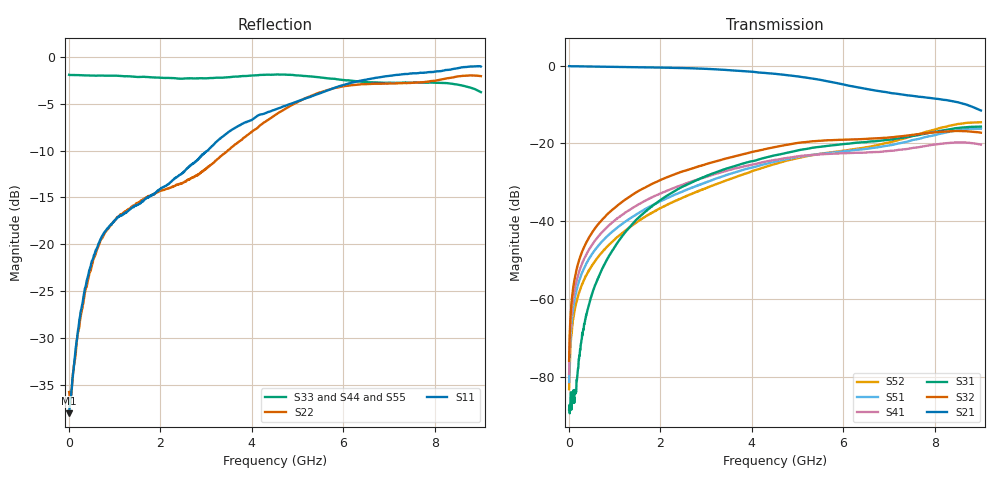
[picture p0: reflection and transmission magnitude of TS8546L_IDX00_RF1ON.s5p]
# GHz S DB R 50
! CMT, SN0916, 25263762, 26.7.0
! Date: 16.07.2026 08:25:07
! Data: Format
! Freq S1.1:dB/Ang S1.2:dB/Ang S1.3:dB/Ang S1.4:dB/Ang S1.5:dB/Ang
!  S2.1:dB/Ang S2.2:dB/Ang S2.3:dB/Ang S2.4:dB/Ang S2.5:dB/Ang
!  S3.1:dB/Ang S3.2:dB/Ang S3.3:dB/Ang S3.4:dB/Ang S3.5:dB/Ang
!  S4.1:dB/Ang S4.2:dB/Ang S4.3:dB/Ang S4.4:dB/Ang S4.5:dB/Ang
!  S5.1:dB/Ang S5.2:dB/Ang S5.3:dB/Ang S5.4:dB/Ang S5.5:dB/Ang
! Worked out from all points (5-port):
!   2001 points, 10 MHz to 9 GHz, reference 50 ohm
!   strongest paths, dB at 10 MHz, 2.257 GHz, 4.505 GHz, 6.753 GHz, 9 GHz:
!     S21: -0.2, -0.6, -2.1, -6.5, -11.6
!     S32: -75.9, -28.2, -21.0, -18.7, -17.3
!     S31: -88.5, -32.7, -23.1, -19.4, -15.7
!     S41: -79.3, -31.7, -24.3, -22.2, -20.3
!     S51: -81.4, -33.5, -24.7, -21.0, -16.3
!     S52: -83.2, -35.2, -25.3, -20.4, -14.6
!   lowest |S11| = -38.1 dB at 10 MHz (marker M1), VSWR 1.03, Z = 51.3 - j0.0589 ohm
!   |S11| at or under -10 dB: start of sweep to 3.035 GHz
